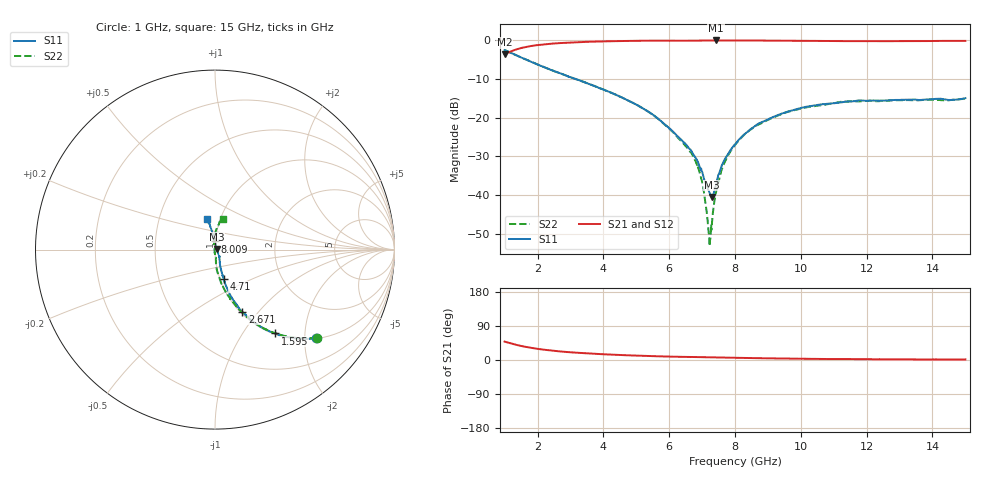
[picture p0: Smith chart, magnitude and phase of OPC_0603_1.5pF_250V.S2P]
! FILE NAME
! DATE 08/20/2012  15:50
! CORRECTED  DATA
# GHz  S  MA  R  50.00
!  FREQ  S11M  S11A  S21M  S21A  S12M  S12A  S22M  S22A
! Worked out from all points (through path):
!   1601 points, 1 GHz to 15 GHz, reference 50 ohm
!   highest |S21| = -0.04 dB at 7.423 GHz (marker M1); lowest = -3.7 dB at 1 GHz (marker M2)
!   group delay of S21, straight-line fit = 6.08 ps
!   lowest |S11| = -40.5 dB at 7.3 GHz (marker M3), VSWR 1.02, Z = 50.8 + j0.427 ohm
!   |S11| at or under -10 dB: 3.15 GHz to end of sweep
!   |S22| runs from -53.3 to -2.5 dB; largest |S21 - S12| = 0.0084
!   S11 on the Smith chart (normalised r, x): 1 GHz: 1.01, -2.27; 1.595 GHz: 1.02, -1.42; 2.671 GHz: 1.02, -0.82; 4.71 GHz: 1.04, -0.35; 8.009 GHz: 0.99, +0.09; 15 GHz: 0.87, +0.31
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1  0.7488 -41.2  0.6557 48.6  0.6554 48.5  0.7496 -40.8
1.595  0.5754 -54.3  0.8099 35.3  0.8098 35.3  0.5756 -53.9
2.67125  0.3771 -66.2  0.9201 22.8  0.9187 22.8  0.3763 -66.8
3.33625  0.2968 -70.2  0.9497 18.4  0.9491 18.4  0.2962 -72.2
4.71  0.1699 -73.7  0.9807 12.5  0.9803 12.5  0.1699 -80.6
5.6725  0.09605 -72.6  0.9904 9.7  0.9901 9.7  0.09563 -86.1
6.145  0.0642 -66.5  0.9891 8.7  0.9885 8.7  0.06282 -86.0
6.73125  0.03335 -52.5  0.9897 7.9  0.989 7.9  0.03103 -87.1
6.985  0.02025 -40.0  0.9922 7.5  0.9914 7.5  0.01571 -97.5
7.0725  0.01546 -31.2  0.9932 7.3  0.9923 7.3  0.009589 -104.6
7.2125  0.01093 -2.6  0.9936 7.1  0.9928 7.1  0.00294 -158.8
7.25625  0.0101 11.0  0.9944 7.0  0.9938 7.0  0.002822 151.4
7.3  0.009397 26.5  0.9946 6.9  0.9942 6.9  0.004296 130.2
7.4225  0.01359 66.8  0.9955 6.6  0.9938 6.6  0.01073 109.2
7.64125  0.02627 83.4  0.9947 6.3  0.9939 6.3  0.02375 102.5
8  0.04518 92.8  0.9944 5.7  0.9932 5.8  0.04416 96.7
8.00875  0.04551 93.0  0.9943 5.7  0.9932 5.7  0.04463 96.3
8.735  0.08485 97.5  0.9924 4.8  0.9915 4.8  0.08206 89.1
9.51375  0.1161 100.5  0.9886 3.9  0.988 3.9  0.1148 85.8
10.33625  0.1419 101.9  0.9837 3.0  0.9826 3.0  0.139 81.7
12.6725  0.1673 108.2  0.972 2.1  0.9717 2.0  0.1657 76.5
15  0.1785 103.9  0.9822 1.5  0.9816 1.5  0.1766 75.3
